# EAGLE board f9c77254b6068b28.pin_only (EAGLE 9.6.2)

Size 157.48 x 50.8 mm. Coordinates in mm from the lower left corner, seen from the top.
Outline: 2.54,50.8 arc90 0,48.26 0,2.54 arc90 2.54,0 154.94,0 arc90 157.48,2.54 157.48,48.26 arc90 154.94,50.8 2.54,50.8
Copper layers (1*16): Top 0.035mm / dielectric 1.5mm / Bottom 0.035mm
Design rules "default": minimum track width 10mil, minimum drill 24mil, track to track 8mil, track to pad 8mil, pad to pad 8mil, via to via 8mil, smd to smd 8mil, copper to edge 40mil, drill to drill 8mil, minimum pad ring 10mil, minimum via ring 8mil, stop-mask expansion 4mil, vias tented up to drill 0mil, thermal gap 10mil
Holes 3.2 mm at 3.81,25.4 153.67,25.4 78.74,25.4

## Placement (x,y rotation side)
U$1  [ADAFRUIT200MIL]  8.38,25.65 270 top

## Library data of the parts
U$1 = adafruit

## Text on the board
tPlace: 1 | 2 | 3 | 4 | 5 | 6 | 7 | 8 | 9 | 10 | 11 | 12 | 13 | 14 | 15 | 16 | 17 | 18 | 19 | 20 | 21 | 22 | 23 | 24 | 25 | 26 | 27 | 28 | 29 | 30 | 31 | 32 | 33 | 34 | 35 | 36 | 37 | 38 | 39 | 40 | 41 | 42 | 43 | 44 | 45 | 46 | 47 | 48 | 49 | 50 | 51 | 52 | 53 | 54 | 55 | 56 | 57 | 58 | 59 | 60 | J | J | I | I | H | H | G | G | F | F | E | E | D | D | C | C | B | B | A | A | 1 | 2 | 3 | 4 | 5 | 6 | 7 | 8 | 9 | 10 | 11 | 12 | 13 | 14 | 15 | 16 | 17 | 18 | 19 | 20 | 21 | 22 | 23 | 24 | 25 | 26 | 27 | 28 | 29 | 30 | 31 | 32 | 33 | 34 | 35 | 36 | 37 | 38 | 39 | 40 | 41 | 42 | 43 | 44 | 45 | 46 | 47 | 48 | 49 | 50 | 51 | 52 | 53 | 54 | 55 | 56 | 57 | 58 | 59 | 60
tDocu: Adafruit Perma-Proto Full Sized Breadboard
tPlaceRed: + | + | + | +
